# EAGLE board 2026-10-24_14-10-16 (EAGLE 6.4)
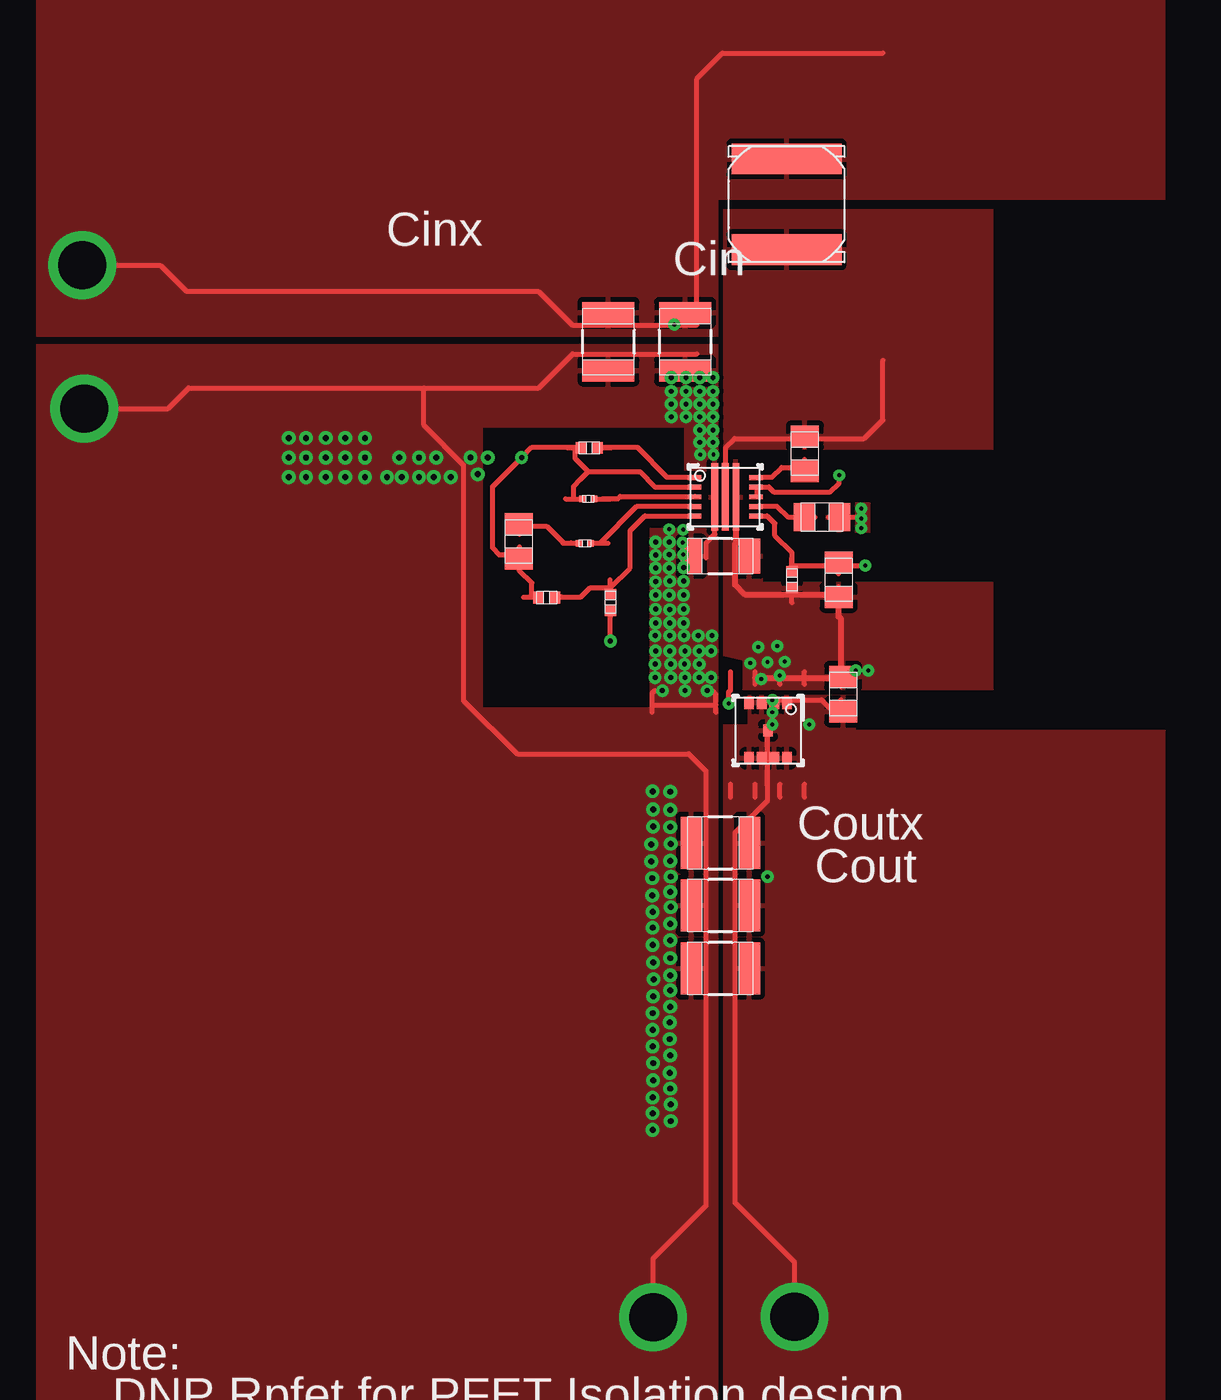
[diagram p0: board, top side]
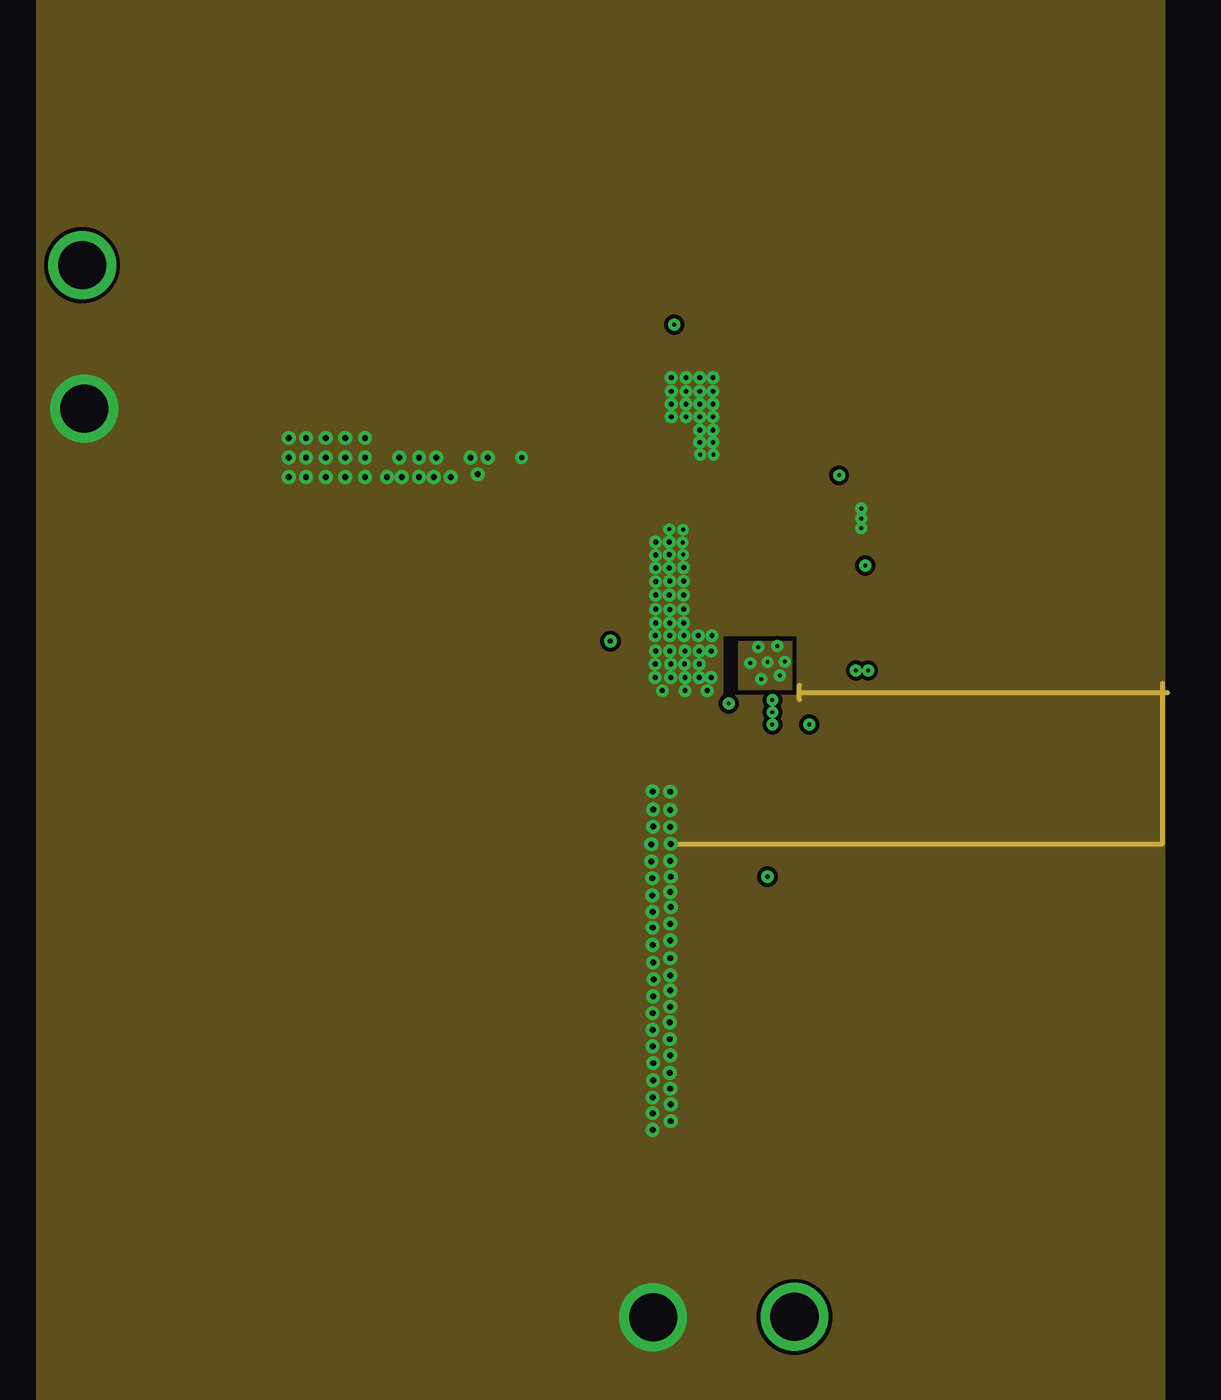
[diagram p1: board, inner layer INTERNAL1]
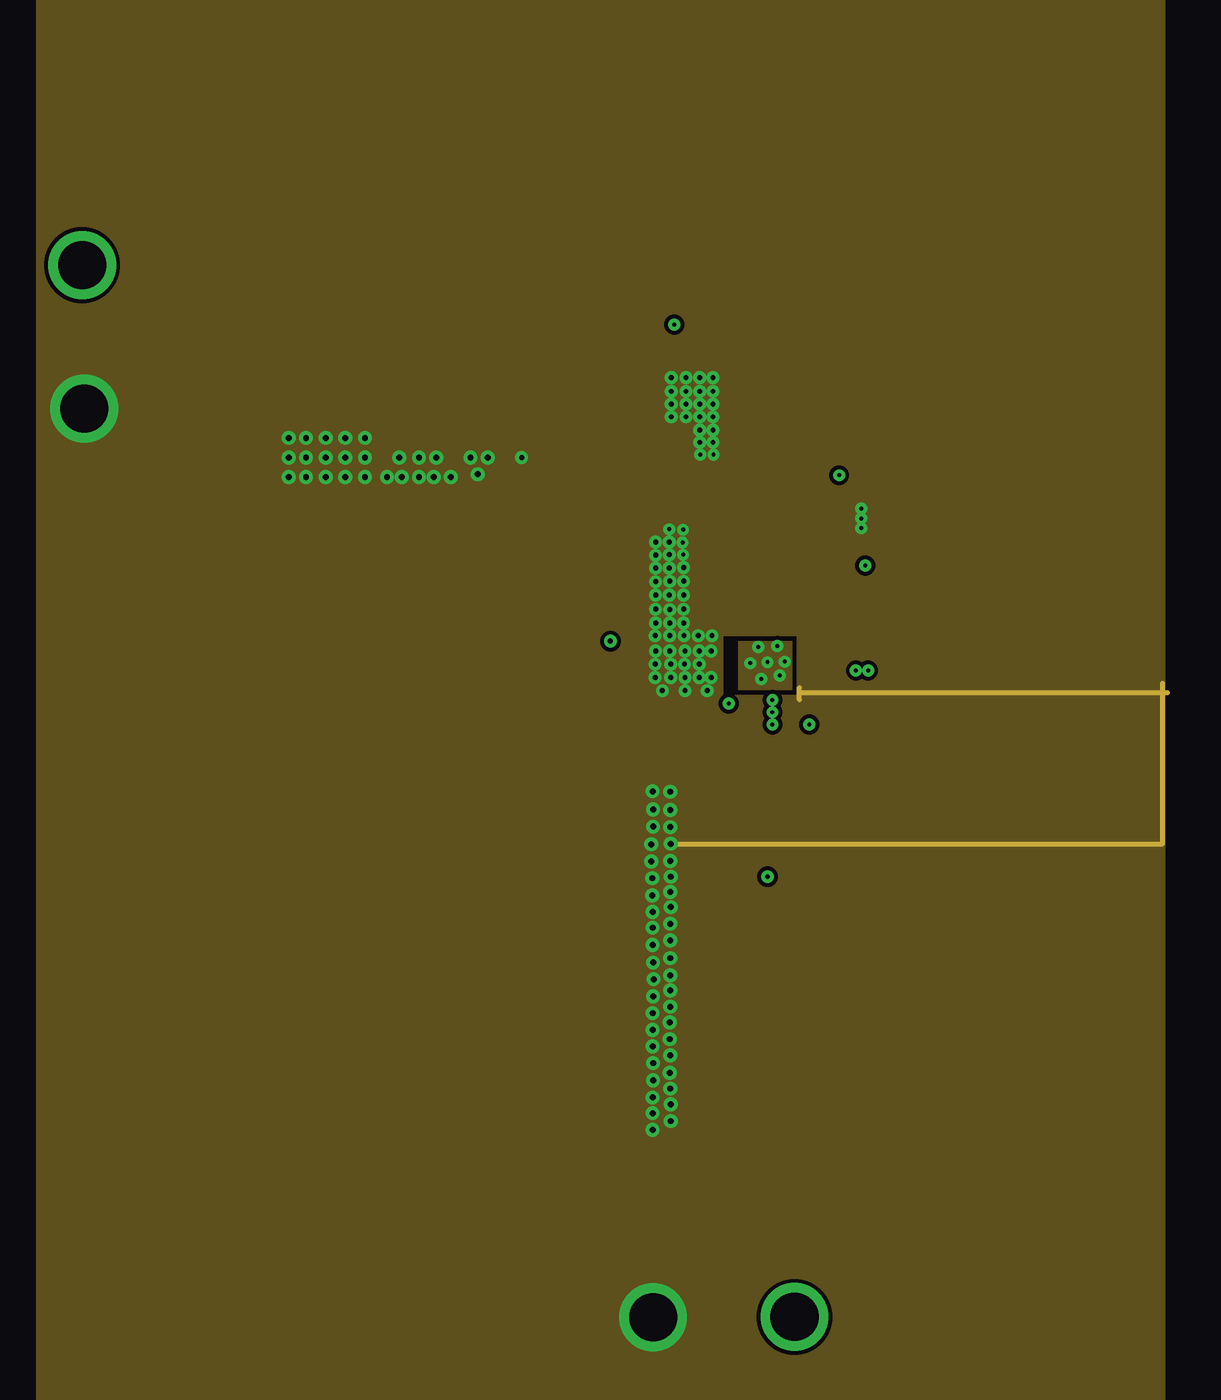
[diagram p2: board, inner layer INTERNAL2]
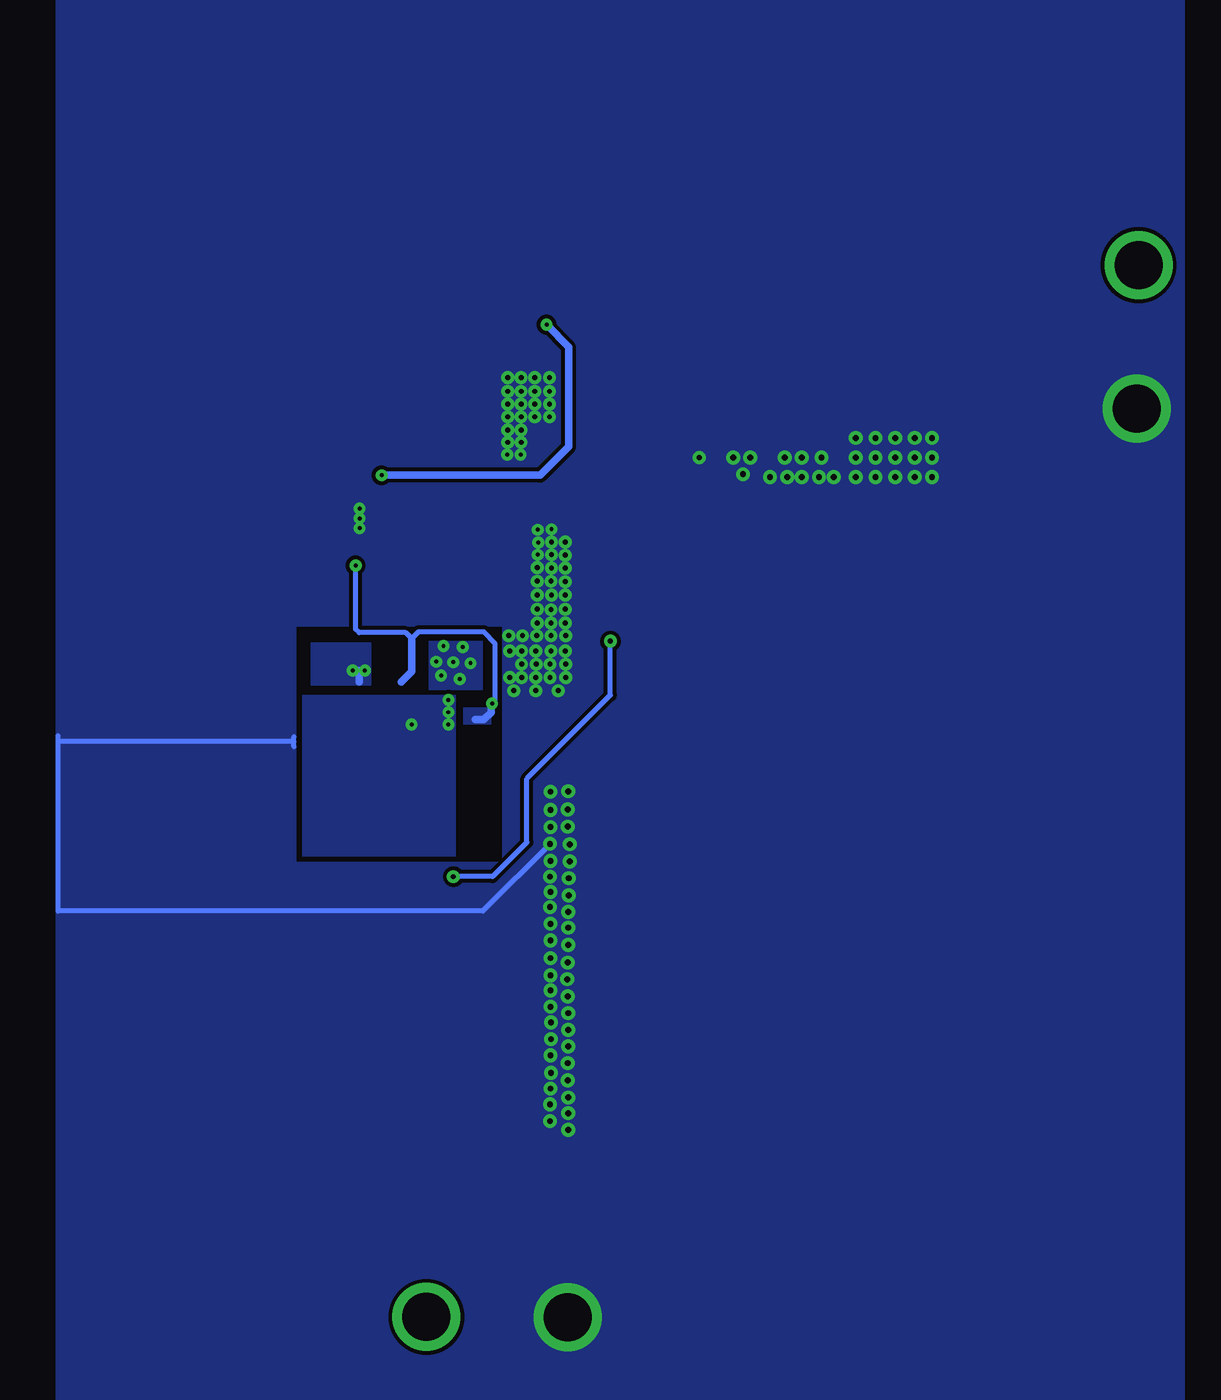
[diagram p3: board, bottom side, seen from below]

No outline drawn. Coordinates in mm, seen from the top.
Copper layers ((1*2)+(15*16)): TOP / INTERNAL1 / layer 15 / BOTTOM

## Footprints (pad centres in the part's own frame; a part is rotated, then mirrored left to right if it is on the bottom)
0805 = smd 1.118 x 1.448: 1 -0.902,0; 2 0.902,0
1210 = smd 1.118 x 2.692: 1 -1.499,0; 2 1.499,0
1206 = smd 1.118 x 1.803: 1 -1.499,0; 2 1.499,0
TP-1502 = drill 0.813 pad 1.651 round: 1 0,0
DG6045C = smd 1.6 x 5.7: 1 -2.35,0; 2 2.35,0
DQG0008A = smd 0.63 x 0.5: 1 -1.435,0.975; 2 -1.435,0.325; 3 -1.435,-0.325; 4 -1.435,-0.975; 5 1.435,-0.975; 6 1.435,-0.325; 7 1.435,0.325; 8 1.435,0.975; 9 0,0
0201 = smd 0.356 x 0.33: 1 -0.292,0; 2 0.292,0
0402 = smd 0.559 x 0.61: 1 -0.419,0; 2 0.419,0
RNW0013A = smd 0.7 x 0.25: 1 -1.6,1; 2 -1.6,0.5; 3 -1.6,0; 4 -1.6,-0.5; 5 -1.6,-1; 9 1.6,-1; 10 1.6,-0.5; 11 1.6,0; 12 1.6,0.5; 13 1.6,1 | smd 0.35 x 3.5: 6 -0.55,0; 7 0,0; 8 0.55,0

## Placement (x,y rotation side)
Cboot  [0805]  66.45,77.77 270 top
Ccomp  [0805]  51.64,73.23 270 top
Cgate  [0805]  68.2,71.25 90 top
Cin_1  [1210]  60.25,83.57 270 top
Cin_2  [1210]  56.29,83.57 270 top
Cout1  [1206]  62.08,72.47 180 top
Cout_1  [1210]  62.08,57.63 180 top
Cout_2  [1210]  62.08,54.38 180 top
Cout_3  [1210]  62.08,51.13 180 top
Cvcc  [0805]  67.34,74.5 0 top
GND  [TP-1502]  58.6,33.05 270 top
GND1  [TP-1502]  29.13,80.09 270 top
L1  [DG6045C]  65.51,90.68 90 top
M3  [DQG0008A]  64.54,63.45 270 top
Rcomp  [0201]  55.07,73.13 180 top
Rfbb  [0402]  53.09,70.33 180 top
Rfbt  [0402]  56.39,70.08 90 top
Rgate  [0402]  65.79,71.25 90 top
Rilim  [0201]  55.24,75.44 180 top
Rpfet  [0805]  68.43,65.33 270 top
Rt  [0402]  55.3,78.08 180 top
U1  [RNW0013A]  62.33,75.54 0 top
VIN  [TP-1502]  29.03,87.53 270 top
VOUT  [TP-1502]  65.89,33.1 270 top

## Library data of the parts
Cboot = ultra-librarian; RefDes: Cboot; Type: 08053C104KAT2A
Ccomp = ultra-librarian; RefDes: Ccomp; Type: CL21C182JBF1PNE
Cgate = ultra-librarian; RefDes: Cgate; Type: C0805C223K5RACTU
Cin_1 Cin_2 Cout_1-Cout_3 = ultra-librarian
Cout1 = ultra-librarian; RefDes: Cout1; Type: C3216X7R1E475K160AC
Cvcc = ultra-librarian; RefDes: Cvcc; Type: MSAST21GAB5475MTNA01
GND = ultra-librarian; RefDes: GND; Type: TP-1502
GND1 = ultra-librarian; RefDes: GND1; Type: TP-1502
L1 = ultra-librarian; RefDes: L1; Type: 1255AY-2R7N=P3
M3 = ultra-librarian; RefDes: M3; Type: CSD25404Q3
Rcomp = ultra-librarian; RefDes: Rcomp; Type: CRCW020144K2FNED
Rfbb = ultra-librarian; RefDes: Rfbb; Type: CRCW040280K6FKED
Rfbt = ultra-librarian; RefDes: Rfbt; Type: CRCW0402732KFKED
Rgate = ultra-librarian; RefDes: Rgate; Type: CRCW0402178KFKED
Rilim = ultra-librarian; RefDes: Rilim; Type: RC0201FR-07162KL
Rpfet = ultra-librarian; RefDes: Rpfet; Type: GRM32ER61E226KE15L
Rt = ultra-librarian; RefDes: Rt; Type: CRCW0402169KFKED
U1 = ultra-librarian; RefDes: U1; Type: TPS61178RNWR
VIN = ultra-librarian; RefDes: VIN; Type: TP-1502
VOUT = ultra-librarian; RefDes: VOUT; Type: TP-1502

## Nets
0: Cboot.2 U1.13
1: Cgate.2 Rgate.2 U1.9
2: Cgate.1 Cout1.1 Rgate.1 Rpfet.1 U1.8
5: Rt.1 U1.1
8: Cin_1.1 Cin_2.1 L1.2 U1.11 U1.12 VIN.1
10: Cboot.1 L1.1 U1.7
11: Rfbb.1 Rfbt.2 U1.5
13: Cout_1.1 Cout_2.1 Cout_3.1 M3.1 M3.2 M3.3 M3.4 M3.5 M3.6 M3.7 M3.8 M3.9 Rfbt.1 Rpfet.2 VOUT.1
14: Ccomp.1 Rcomp.2
18: Ccomp.2 Cin_1.2 Cin_2.2 Cout1.2 Cout_1.2 Cout_2.2 Cout_3.2 Cvcc.2 GND1.1 GND.1 Rfbb.2 Rilim.2 Rt.2 U1.2 U1.6
19: Cvcc.1 U1.10
24: Rcomp.1 U1.4
27: Rilim.1 U1.3

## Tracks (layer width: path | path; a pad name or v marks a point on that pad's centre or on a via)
0
  TOP 0.254: 63.96,76.56 64.75,76.56 65.25,77.06 66.45,77.06 | 66.43,76.63 66.43,77.47
1  (via drill 0.2 pad 0.46, 0.2 pad 0.48)
  TOP 0.254: 63.96,74.55 64.49,74.55 64.9,74.17 64.9,73.53 65.79,72.64 65.79,71.98 68.2,71.98 | 68.2,71.98 | 68.2,71.98 v69.57,71.98 | v62.51,64.85 62.51,65.43 62.61,65.53 62.61,66.17 | 65.77,71.55 65.77,72.39 | 68.19,71.55 68.19,72.39 | 62.61,65.84 62.61,66.5
  BOTTOM 0.254: v69.57,71.98 69.57,68.68 69.39,68.5 66.98,68.5 66.67,68.2 66.32,68.56 62.92,68.56 62.36,67.94 62.36,65.02 v62.51,64.85 62.59,64.77
  BOTTOM 0.381: 66.67,68.2 66.67,66.5 67.21,65.96 | 63.37,64.01 62.94,64.01 62.56,64.39 62.56,64.75
  pour BOTTOM: 64.01,64.64 64.01,63.75 62.56,63.75 62.56,64.64
2  (via drill 0.2 pad 0.48)
  TOP 0.254: 65.77,70.05 65.77,70.89 | 68.19,70.05 68.19,70.89 | 68.31,65.71 68.31,66.55 | 66.42,65.84 66.42,66.5 | 65.15,65.84 65.15,66.5 | 63.88,65.84 63.88,66.5 | 65.79,70.48
  TOP 0.305: 62.89,75.56 62.89,73.15 62.84,73.1 62.84,72.39 62.84,70.99 63.35,70.48 65.79,70.48 68.2,70.48 68.2,69.34 68.33,69.22 68.33,66.14 68.3,66.17 66.42,66.17 65.15,66.17 63.88,66.17
  BOTTOM 0.381: 69.39,66.55 v69.72,66.55 | v69.09,66.55 69.39,66.55 | 69.39,65.96 69.39,66.55
  other vias: 64.03,67.77 64.19,66.12 65.02,67.82 65.15,66.29 64.52,66.98 65.41,67.01 63.63,66.93
  pour TOP: 62.23,67.31 63.25,67.06 63.25,65.53 76.2,65.53 76.2,71.12 64.26,71.12 64.26,73.38 63.25,73.38 63.25,77.47 62.74,77.47 62.74,73.38 62.23,73.38
  pour BOTTOM: 62.99,65.53 65.79,65.53 65.79,68.07 62.99,68.07
  pour BOTTOM (rank 3): 68.76,65.79 71.88,65.79 71.88,68 68.76,68
  pour INTERNAL2 (rank 3): 62.99,68.07 65.79,68.07 65.79,65.53 62.99,65.53
  pour INTERNAL1 (rank 4): 62.99,68.07 65.79,68.07 65.79,65.53 62.99,65.53
5
  TOP 0.254: 56.06,78.11 57.78,78.11 | 57.78,78.11 | 57.78,78.11 59.31,76.56 60.76,76.56 | 55.63,78.09 56.46,78.09
8  (via drill 0.2 pad 0.46, 2.49 pad 3.48)
  TOP 0.203: 63.96,75.56 63.96,76.05
  TOP 0.254: v68.22,76.66 68.22,76.25 67.74,75.79 64.85,75.79 64.59,76.05 63.96,76.05 | v29.06,87.53 33.1,87.53 34.44,86.18 46.74,86.18 52.65,86.18 54.41,84.43 60.86,84.43 60.86,97.18 62.18,98.5 70.48,98.5
  BOTTOM 0.381: v68.22,76.66 60.02,76.66 58.55,78.13 58.55,83.29 v59.69,84.45
  pour TOP (rank 6): 26.67,110.74 85.09,110.74 85.09,90.93 61.98,90.93 61.98,83.82 26.67,83.82
10
  TOP 0.254: 62.36,75.56 62.36,78.11 62.81,78.56 66.45,78.56 69.52,78.56 70.48,79.5 70.48,82.6 | 66.43,78.13 66.43,78.97
  pour TOP: 62.23,77.98 62.23,90.42 76.2,90.42 76.2,77.98
11
  TOP 0.254: 53.82,70.36 54.86,70.36 55.35,70.84 56.39,70.84 57.4,71.86 57.4,73.79 58.17,74.55 60.76,74.55 | 56.38,70.41 56.38,71.25 | 53.39,70.34 54.23,70.34
13  (via drill 0.2 pad 0.46, 0.25 pad 0.51, 2.49 pad 3.48)
  TOP 0.254: 62.84,55.85 | 62.84,55.85 62.84,58.17 64.52,59.82 64.52,62.03 64.52,63.5 v64.77,63.75 v64.77,64.39 v64.77,65.02 67.31,65.02 67.67,64.64 68.33,64.64 | v65.91,33.1 65.91,35.92 62.84,38.99 62.84,55.85 | v56.39,68.07 56.39,69.34 | 56.38,68.91 56.38,69.75 | 68.31,64.21 68.31,65.05 | 62.61,59.99 62.61,60.66 | 63.88,59.99 63.88,60.66 | 65.15,59.99 65.15,60.66 | 66.42,59.99 66.42,60.66 | 64.5,60.6 64.5,63.48
  BOTTOM 0.254: v64.52,55.88 62.48,55.88 60.71,57.66 60.71,60.96 56.39,65.28 v56.39,68.07
  other vias: 66.67,63.75
  pour TOP (rank 5): 63.5,65.28 63.5,63.75 62.23,63.75 62.23,26.67 85.09,26.67 85.09,63.47 69.09,63.47 69.09,65.28
  pour BOTTOM (rank 2): 64.39,65.28 64.39,56.92 72.34,56.92 72.34,65.28
14
  TOP 0.254: 54.36,73.15 53.98,73.15 53.09,74.02 51.66,74.02 | 51.68,73.61 51.68,74.45 | 53.92,73.14 54.76,73.14
18  (via drill 0.2 pad 0.46, 0.25 pad 0.51, 0.3 pad 0.61, 2.49 pad 3.48)
  TOP 0.254: 46.74,81.18 34.57,81.18 33.5,80.11 v29.16,80.11 | 58.55,64.39 58.55,64.77 | 58.55,64.77 58.55,65.38 58.67,65.51 v59.08,65.51 | 61.85,64.39 61.85,64.77 | 58.55,64.77 61.85,64.77 | 61.34,58.17 61.34,61.32 60.45,62.23 51.56,62.23 48.79,64.97 48.79,77.17 46.74,79.25 46.74,81.18 | 61.34,58.17 | 61.34,58.17 61.34,55.85 61.34,38.86 58.6,36.12 v58.6,33.07 | 68.07,74.5 69.29,74.5 v69.37,74.42 | 61.34,72.39 61.34,73.15 61.8,73.61 61.8,75.56 | 55.24,76.83 57.91,76.83 58.67,76.05 60.86,76.05 | 61.85,64.77 61.85,65.3 61.65,65.51 v61.39,65.51 | 46.74,81.18 52.68,81.18 54.43,82.93 60.86,82.93 | 55.24,76.83 54.86,76.45 54.48,76.07 54.48,75.44 | 55.24,76.83 54.56,77.52 54.56,78.11 52.32,78.11 v51.79,77.57 50.29,76.07 50.29,72.9 50.62,72.54 51.66,72.54 51.66,71.73 52.32,71.09 52.32,70.36 | 51.68,72.11 51.68,72.95 | 51.89,70.34 52.73,70.34 | 54.08,75.42 54.91,75.42 | 54.13,78.09 54.97,78.09 | 67.67,74.49 68.5,74.49
  INTERNAL1 0.254: 84.96,65.41 85.22,65.41 | 66.17,65.41 84.96,65.41 | 66.17,65.05 66.17,65.41 | 66.17,65.41 66.17,65.79 | 84.96,65.41 84.96,65.89 | 84.96,65.41 84.96,57.58 v59.51,57.58 59.49,57.58
  INTERNAL2 0.254: 84.96,65.41 85.22,65.41 | 66.17,65.41 84.96,65.41 | 66.17,65.05 66.17,65.41 | 84.96,65.41 84.96,57.58 v59.51,57.58 | 84.96,65.41 84.96,65.89 | v59.51,57.58 | 66.17,65.41 66.17,65.66
  BOTTOM 0.254: 72.77,62.87 72.77,63.12 | 72.77,62.61 72.77,62.87 | 84.96,62.87 84.96,63.17 | 84.96,62.87 84.96,54.1 62.99,54.1 v59.51,57.58 | 72.77,62.87 84.96,62.87 | 59.49,57.58
  other vias: 60.3,81.71 60.3,79.68 60.25,65.51 60.17,71.17 60.25,67.56 50.04,77.57 39.75,77.57 41.66,77.57 43.69,77.57 44.83,76.56 45.59,76.56 47.24,76.56 59.44,72.54 59.44,71.86 58.72,70.46 61.59,66.19 59.44,70.46 59.49,60.27 59.49,58.45 59.49,56.69 59.51,55.88 59.51,54.31 59.49,52.58 59.49,51.66 59.49,49.99 59.46,48.34 59.46,47.47 59.49,46.63 59.46,45.72 59.51,44.09 58.57,60.3 58.6,58.47 58.5,57.56 58.5,56.67 58.55,55.8 58.57,54.05 58.57,52.35 58.62,50.57 58.6,49.68 58.57,47.96 58.6,46.23 58.6,45.34 58.57,44.45 58.57,43.64 59.46,69.01 58.72,69.72 58.72,69.01 58.7,68.35 59.46,68.35 59.51,66.19 58.7,66.88 60.99,66.19 60.99,66.88 46.48,76.56 40.64,76.56 42.67,76.56 40.64,78.59 42.67,78.59 49.53,76.71 60.93,68.35 58.72,72.52 58.72,71.86 59.44,73.86 59.54,81 59.54,80.34 61.65,68.35 61.01,78.99 61.7,78.36 61.01,78.36 61.7,78.99 61.01,81 61.7,80.34 61.7,81 61.01,80.34 69.37,74.93 69.37,73.91 40.64,77.57 42.67,77.57 45.47,77.57 47.37,77.57 46.48,77.57 49.15,77.57 59.46,71.17 58.72,71.15 59.44,73.2 58.72,73.2 59.54,79.68 59.54,81.71 61.7,79.68 61.72,77.72 61.01,79.68 61.04,77.72 61.01,81.71 61.7,81.71 39.75,76.56 41.66,76.56 43.69,76.56 39.75,78.59 41.66,78.59 43.69,78.59 48.13,76.56 59.49,44.91 59.51,43.23 58.57,47.09 58.57,42.77 59.49,55.09 59.49,53.44 59.49,50.77 59.49,49.15 58.55,54.91 58.57,53.24 58.6,51.44 58.57,48.82 59.49,59.33 58.6,59.36 60.25,66.19 59.51,66.88 58.7,66.19 58.72,67.56 59.46,69.7 60.15,73.84 60.3,80.34 60.3,81 59.46,67.56 60.99,67.56 61.59,67.56 60.22,66.88 60.17,69.01 60.2,68.35 60.17,70.46 60.17,69.72 60.17,71.88 60.12,73.18 60.15,72.54
  pour TOP (rank 6): 58.42,64.64 49.78,64.64 49.78,79.12 60.2,79.12 60.2,76.83 61.47,76.83 61.47,73.91 58.42,73.91 58.42,64.9 61.98,64.9 61.98,83.44 26.67,83.44 26.67,26.67 61.98,26.67 61.98,64.64
  pour TOP: 67.54,75.23 69.82,75.23 69.82,73.69 67.54,73.69
  pour BOTTOM (rank 2): 72.64,56.64 72.64,62.74 85.09,62.74 85.09,56.26 85.09,26.67 26.67,26.67 26.67,110.74 85.09,110.74 85.09,62.99 72.64,62.99 72.64,68.83 61.98,68.83 61.98,56.64
  pour INTERNAL2 (rank 4): 26.67,110.74 26.67,26.67 85.09,26.67 85.09,65.28 62.23,65.28 62.23,68.33 66.04,68.33 66.04,65.53 85.09,65.53 85.09,110.74
  pour INTERNAL1 (rank 5): 26.67,110.74 26.67,26.67 85.09,26.67 85.09,65.28 62.23,65.28 62.23,68.33 66.04,68.33 66.04,65.53 85.09,65.53 85.09,110.74
19
  TOP 0.254: 63.96,75.06 65,75.06 65.58,74.5 66.57,74.5 | 66.14,74.49 66.98,74.49
24
  TOP 0.254: 55.85,73.15 57.76,75.06 60.76,75.06 | 55.42,73.14 56.26,73.14
27
  TOP 0.254: 60.76,75.56 56.9,75.56 56.77,75.44 55.98,75.44 | 55.58,75.42 56.41,75.42

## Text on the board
ASSYNOTES: Cinx | Cin | Coutx | Cout | Note: | DNP Rpfet for PFET Isolation design.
